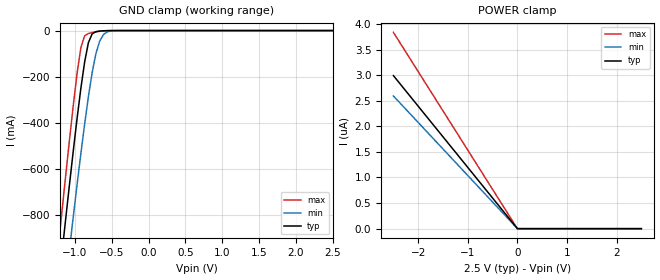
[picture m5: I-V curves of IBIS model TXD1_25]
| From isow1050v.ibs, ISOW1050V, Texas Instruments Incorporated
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|   TXD1_25 Model
[Model] TXD1_25
Model_type Input
Polarity   Non-Inverting
Enable   Active-High
Vinl =  0.750V
Vinh =  1.750V
C_comp   1.300pF   1.100pF   1.500pF
[Model Spec]
Vinh   1.750V   1.575V   1.925V
Vinl   0.750V   0.675V   0.825V
[Temperature Range]   27.000   0.150k   -55.000
[Voltage Range]   2.500V   2.250V   2.750V
[POWER Clamp Reference]   2.500V   2.250V   2.750V
[GND Clamp Reference]   0.0V   0.0V   0.0V
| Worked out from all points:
|   GND clamp passes 1 mA (typ) near -0.62 V on its own axis
[GND_clamp]
|Voltage   I(typ)   I(min)   I(max)
-2.5V     -4.871A    -4.741A    -5.007A
-1.225V   -1.114A    -1.38A     -938.7mA
-1.174V   -962.2mA   -1.234A    -779.8mA
-1.123V   -811.8mA   -1.089A    -623.1mA
-1.072V   -663.9mA   -945.7mA   -469.8mA
-1.021V   -519.6mA   -805mA     -322mA
-919mV    -250.7mA   -533.8mA   -73.8mA
-817mV    -52.7mA    -287.5mA   -12.67mA
-715mV    -4.693mA   -99.88mA   -5.686mA
-664mV    -2.077mA   -45.91mA   -3.219mA
-562mV    -351uA     -5.395mA   -481.8uA
2.5V      0A         0A         -383.5nA
[POWER_clamp]
|Voltage   I(typ)   I(min)   I(max)
-2.5V     2.99uA     2.593uA    3.835uA
-50mV     59.85nA    53.58nA    76.75nA
1mV       0A         705.1pA    0A
2.5V      0A         0A         0A
